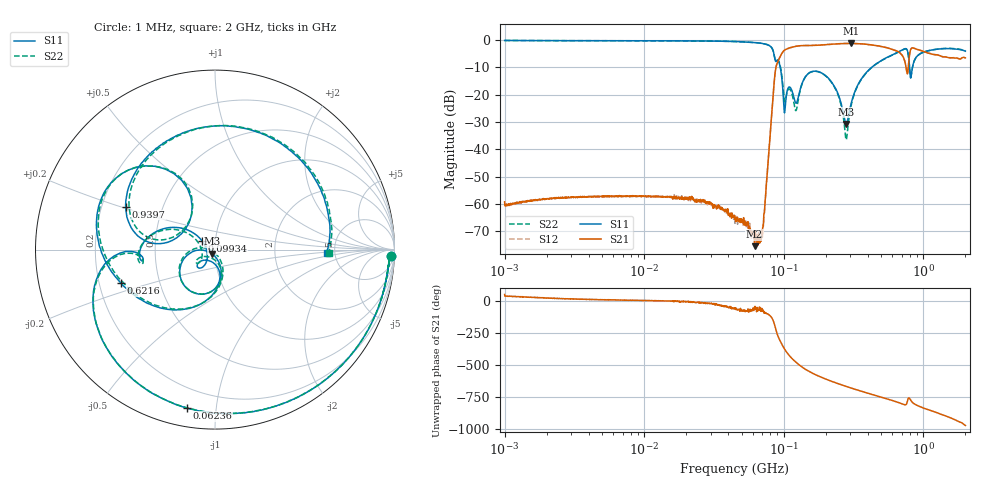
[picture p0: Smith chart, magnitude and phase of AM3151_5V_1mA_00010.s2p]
! Date/Time: Fri Jun 26 10:28:42 2020
! Network Analyzer:  Rev:
! Sweep from 1000000.0 to 2000000000.0, 1601 Points ! Power Supply: 0 V, 0 A
# HZ S DB R 50
!freq MagS11 AngS11 MagS21 AngS21 MagS12 AngS12 MagS22 AngS22
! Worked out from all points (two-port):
!   1601 points, 1 MHz to 2 GHz, reference 50 ohm
!   highest |S21| = -1.26 dB at 301.9 MHz (marker M1); lowest = -75.5 dB at 61.77 MHz (marker M2)
!   |S21| within 3 dB of the highest: 98.87 MHz to 657.7 MHz (558.8 MHz wide, 148 % of centre); 803 MHz to 1.012 GHz (208.8 MHz wide, 23 % of centre)
!   lowest |S11| = -30.8 dB at 279.8 MHz (marker M3), VSWR 1.06, Z = 48.3 - j2.25 ohm
!   |S11| at or under -10 dB: 94.36 MHz to 426.5 MHz (332.1 MHz wide, 128 % of centre); 795.9 MHz to 835.6 MHz (39.68 MHz wide, 4.86 % of centre)
!   |S22| runs from -36.6 to -0.2 dB; largest |S21 - S12| = 0.0097
!   S11 on the Smith chart (normalised r, x): 1 MHz: 24, -42; 62.36 MHz: 0.09, -0.83; 99.34 MHz: 0.86, +0.08; 621.6 MHz: 0.29, -0.16; 939.7 MHz: 0.30, +0.21; 2 GHz: 4.30, -0.24
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1000000  -0.17 -2.1  -59.26 50.4  -60.39 38.1  -0.18 -2.1
3555161  -0.26 -5.5  -57.44 14.6  -57.69 14.1  -0.26 -5.5
1.263916e7  -0.30 -18.5  -57.39 1.4  -57.15 1.6  -0.30 -18.5
4.493426e7  -0.58 -68.0  -64.93 -53.6  -66.02 -68.4  -0.59 -68.0
6.177434e7  -0.92 -98.8  -75.49 -46.9  -70.18 -40.5  -0.95 -98.8
6.23641e7  -0.95 -100.1  -70.27 -56.2  -73.30 -52.6  -0.96 -100.1
6.989562e7  -1.25 -117.4  -69.48 -59.0  -72.41 -91.9  -1.26 -117.3
8.655485e7  -7.15 -177.9  -12.26 160.7  -12.25 160.7  -7.16 -176.5
9.250714e7  -8.29 170.8  -6.91 65.7  -6.91 65.7  -7.99 173.7
9.933959e7  -21.19 146.0  -4.13 -0.1  -4.14 -0.1  -18.61 152.9
1.173094e8  -20.43 -139.8  -2.51 -100.8  -2.50 -100.8  -22.17 -149.8
1.589914e8  -11.57 -110.3  -2.00 157.8  -1.99 157.7  -11.60 -110.6
2.292112e8  -16.81 -170.9  -1.51 85.1  -1.51 85.0  -17.01 -176.1
2.798254e8  -30.76 -126.5  -1.29 52.4  -1.30 52.4  -36.58 -128.2
3.019241e8  -23.79 -74.4  -1.26 40.4  -1.27 40.5  -24.58 -62.9
5.652395e8  -6.09 -145.7  -3.04 -49.7  -3.02 -49.5  -6.14 -147.0
6.215777e8  -5.07 -160.5  -3.70 -63.1  -3.70 -63.1  -5.15 -162.2
7.624488e8  -3.49 140.7  -12.05 -77.2  -12.05 -77.0  -3.66 137.6
8.226611e8  -12.28 167.9  -3.02 -65.1  -3.01 -65.1  -12.21 163.7
9.397004e8  -5.16 154.2  -3.70 -104.3  -3.71 -104.3  -5.20 150.7
1.393896e9  -3.18 81.4  -6.18 -171.8  -6.18 -172.0  -3.13 78.1
2e9  -4.10 -1.6  -6.53 107.1  -6.69 106.7  -3.97 -1.6
